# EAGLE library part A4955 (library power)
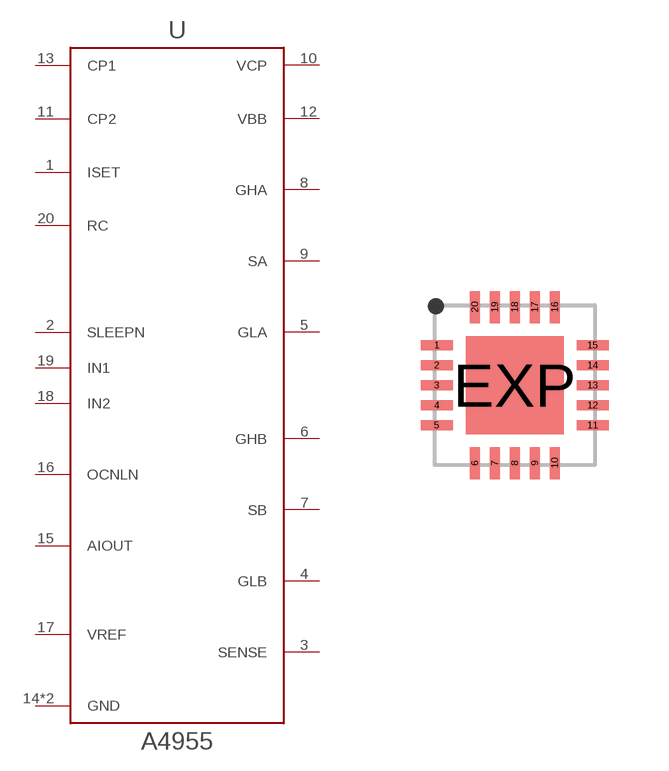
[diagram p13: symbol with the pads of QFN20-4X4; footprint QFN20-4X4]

Designator prefix -

## A4955QFN20  [QFN20-4X4]
1  ISET
2  SLEEPN
3  SENSE
4  GLB
5  GLA
6  GHB
7  SB
8  GHA
9  SA
10  VCP
11  CP2
12  VBB
13  CP1
14  GND
15  AIOUT
16  OCNLN
17  VREF
18  IN2
19  IN1
20  RC
EXP  GND

## Footprint QFN20-4X4 (pad centres in mm)
QFN 20 4 x 4 mm
smd 0.8 x 0.25: 1 -1.95,1; 2 -1.95,0.5; 3 -1.95,0; 4 -1.95,-0.5; 5 -1.95,-1; 11 1.95,-1; 12 1.95,-0.5; 13 1.95,0; 14 1.95,0.5; 15 1.95,1
smd 0.25 x 0.8: 6 -1,-1.95; 7 -0.5,-1.95; 8 0,-1.95; 9 0.5,-1.95; 10 1,-1.95; 16 1,1.95; 17 0.5,1.95; 18 0,1.95; 19 -0.5,1.95; 20 -1,1.95
smd 2.45 x 2.45: EXP 0,0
